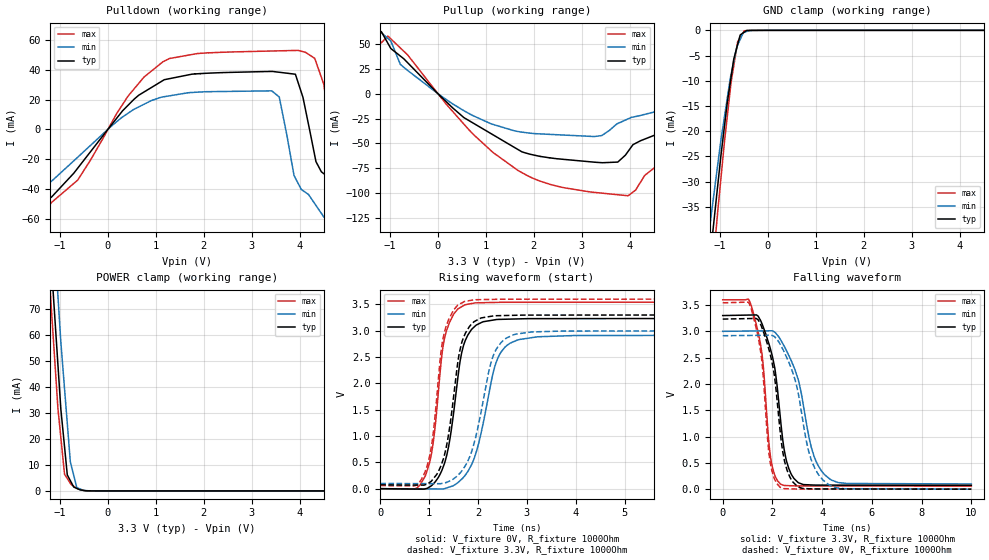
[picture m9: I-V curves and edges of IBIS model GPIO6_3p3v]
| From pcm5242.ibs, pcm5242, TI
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|   Model
[Model]   GPIO6_3p3v
Model_type   I/O
Polarity   Non-Inverting
Enable   Active-Low
Vinl = 0.99
Vinh = 2.31
Vmeas = 1.65
Vref = 0
Cref = 1pF
Rref = 1000000
|   typ   min   max
C_comp   1.371pF   1.337pF   1.391pF
[Voltage Range]   3.3   3   3.6
[Temperature Range]   27   105   -25
[Pullup Reference]   3.3   3   3.6
[Pulldown Reference]   -0   -0   -0
[Power Clamp Reference]   3.3   3   3.6
[GND Clamp Reference]   -0   -0   -0
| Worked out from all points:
|   slope of the pulldown table from 0 to 0.495 V, typ, clamps not added: 26.6 ohm
|   slope of the pullup table from 0 to 0.495 V, typ, clamps not added: 22.4 ohm
|   GND clamp passes 1 mA (typ) near -0.58 V on its own axis
|   POWER clamp passes 1 mA (typ) near -0.65 V on its own axis
|   falling waveform, V_fixture 3.3V, R_fixture 1000Ohm: 20-80 % time 561ps typ, 862ps min, 416ps max; typ from 3.3 V to 0.073 V
|   rising waveform, V_fixture 0V, R_fixture 1000Ohm: 20-80 % time 304ps typ, 423ps min, 255ps max; typ from 0 V to 3.23 V
|   rising waveform, V_fixture 3.3V, R_fixture 1000Ohm: 20-80 % time 303ps typ, 414ps min, 255ps max; typ from 0.073 V to 3.3 V
|   falling waveform, V_fixture 0V, R_fixture 1000Ohm: 20-80 % time 544ps typ, 819ps min, 405ps max; typ from 3.23 V to 0 V
[Pulldown]
|   Voltage   I(typ)   I(min)   I(max)
-3.3V     -1.19mA    -1.068mA   -1.279mA
-3.13V    -56.53mA   -55.88mA   -56.93mA
-2.96V    -65.45mA   -64.53mA   -66.01mA
-1.97V    -54.07mA   -42.32mA   -64.09mA
2.049V    37.7mA     25.31mA    51.39mA
3.573V    38.38mA    21.74mA    52.79mA
3.967V    31.36mA    -36.34mA   53.09mA
4.503V    -29.82mA   -58.92mA   30.09mA
4.824V    -61.07mA   -59.68mA   -27.47mA
6.399V    -64.47mA   -62.21mA   -65.36mA
6.41V     -33.93mA   -62.22mA   -26.95mA
6.6V      774.6mA    899.5mA    659.9mA
[GND Clamp]
|   Voltage   I(typ)   I(min)   I(max)
-3.3V     -527.4mA   -490.8mA   -553.6mA
-1.376V   -61.94mA   -52.32mA   -72.28mA
-1.178V   -42.72mA   -36.47mA   -50.11mA
-1.04V    -30.42mA   -26.36mA   -35.52mA
-903.2mV  -18.92mA   -17.07mA   -22mA
-845.4mV  -14.35mA   -13.44mA   -17.07mA
-765.8mV  -9.242mA   -8.708mA   -10.28mA
-711mV    -5.727mA   -6.208mA   -7.074mA
-628.5mV  -2.773mA   -2.891mA   -2.254mA
-576.6mV  -915.3uA   -1.812mA   -1.435mA
-491.1mV  -356.1uA   -386.2uA   -88.49uA
6.6V      0A         0A         0A
[Pullup]
|   Voltage   I(typ)   I(min)   I(max)
-3.3V     618.1uA    488.4uA    720.8uA
-3.13V    56.63mA    56.35mA    56.84mA
-2.96V    65.79mA    65.46mA    66.04mA
-1.376V   64.46mA    63.29mA    66.01mA
1.111V    -40.26mA   -30.36mA   -57.44mA
3.967V    -57.96mA   -25.3mA    -102.6mA
4.889V    -31.47mA   -7.957mA   -60.26mA
5.395V    15.5mA     50.91mA    -41.01mA
5.613V    49.25mA    56.22mA    -10.62mA
5.998V    55.5mA     58.55mA    51.16mA
6.403V    62.09mA    60.55mA    52.16mA
6.6V      -529.1mA   -589.3mA   -458.7mA
[POWER Clamp]
|   Voltage   I(typ)   I(min)   I(max)
-3.3V     774.1mA    800.5mA    758.1mA
-1.376V   148.1mA    176.3mA    130.9mA
-1.178V   87.23mA    115.2mA    70.27mA
-1.04V    48.6mA     75.07mA    31.77mA
-979.8mV  31.54mA    57.35mA    20.58mA
-903.2mV  17.07mA    39.47mA    6.438mA
-845.4mV  6.179mA    26mA       4.774mA
-781.8mV  3.962mA    11.17mA    2.942mA
-711mV    1.49mA     5.978mA    1.81mA
-646.4mV  967uA      1.248mA    1.02mA
-576.6mV  400.8uA    714.3uA    526.4uA
6.6V      0A         0A         0A
[Ramp]
R_load = 1000
|   typ   min   max
dV/dt_r   1.93982/3.03612e-10   1.74984/4.22975e-10   2.12533/2.54052e-10
dV/dt_f   1.93633/5.57495e-10   1.74079/8.56863e-10   2.12492/4.13507e-10
[Falling Waveform]
V_fixture = 3.3V
V_fixture_min = 3V
V_fixture_max = 3.6V
R_fixture = 1000Ohm
C_fixture = 0F
|   Time   V(typ)   V(min)   V(max)
0s        3.3V       3V         3.6V
1.148ns   3.31V      3.006V     3.487V
1.586ns   3.138V     3.009V     2.55V
1.897ns   2.704V     3.01V      703.5mV
2.325ns   1.325V     2.843V     96.07mV
2.543ns   580.2mV    2.653V     68.48mV
2.864ns   204mV      2.32V      63.44mV
3.666ns   78.23mV    636mV      60.9mV
4.312ns   76.92mV    191mV      60.65mV
10ns      72.79mV    98.68mV    58.46mV
[Rising Waveform]
V_fixture = 0V
V_fixture_min = 0V
V_fixture_max = 0V
R_fixture = 1000Ohm
C_fixture = 0F
|   Time   V(typ)   V(min)   V(max)
0s        1.823nV    31.53nV    1.041nV
909.6ps   -5.708mV   -3.811mV   221mV
1.08ns    86.37mV    -4.525mV   854.2mV
1.195ns   225.2mV    -5.005mV   1.904V
1.354ns   616.5mV    12.99mV    2.998V
1.728ns   2.787V     244.4mV    3.489V
1.978ns   3.114V     742.1mV    3.529V
2.381ns   3.212V     2.426V     3.537V
2.797ns   3.223V     2.819V     3.539V
10ns      3.233V     2.916V     3.542V
[Rising Waveform]
V_fixture = 3.3V
V_fixture_min = 3V
V_fixture_max = 3.6V
R_fixture = 1000Ohm
C_fixture = 0F
|   Time   V(typ)   V(min)   V(max)
0s        72.78mV    98.58mV    58.46mV
844ps     67.82mV    95.74mV    180.9mV
1.034ns   134mV      95.1mV     735.4mV
1.169ns   292.1mV    94.64mV    1.873V
1.338ns   737mV      115mV      3.056V
1.711ns   2.888V     393.1mV    3.549V
1.925ns   3.174V     882.3mV    3.587V
2.306ns   3.279V     2.511V     3.594V
2.725ns   3.291V     2.922V     3.597V
10ns      3.3V       3V         3.6V
[Falling Waveform]
|Gnd
V_fixture = 0V
V_fixture_min = 0V
V_fixture_max = 0V
R_fixture = 1000Ohm
C_fixture = 0F
|   Time   V(typ)   V(min)   V(max)
0s        3.233V     2.917V     3.542V
1.148ns   3.244V     2.923V     3.424V
1.561ns   3.09V      2.925V     2.493V
1.939ns   2.51V      2.927V     438.6mV
2.306ns   1.122V     2.759V     37.46mV
2.495ns   516mV      2.584V     9.493mV
2.822ns   136.1mV    2.212V     4.985mV
3.556ns   5.593mV    565.3mV    2.217mV
4.241ns   3.925mV    93.5mV     1.981mV
10ns      4.985uV    86.51uV    916.2nV
